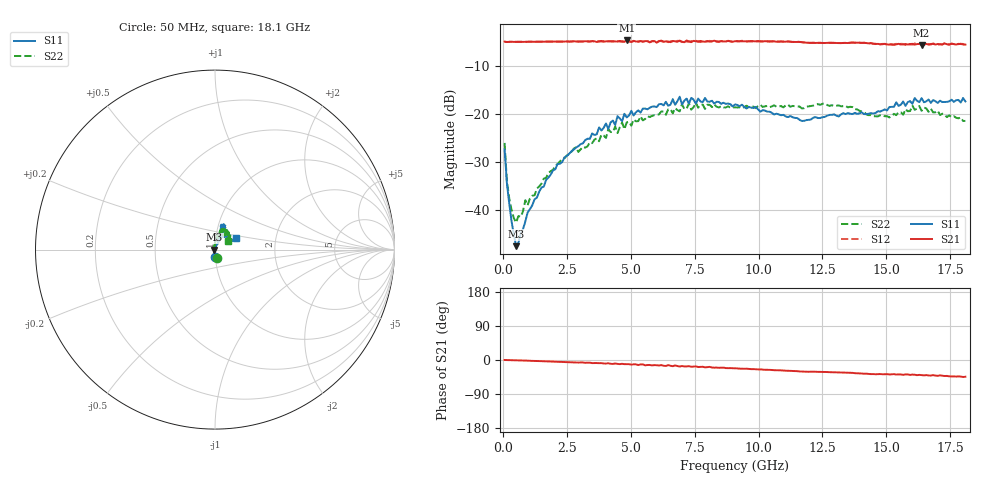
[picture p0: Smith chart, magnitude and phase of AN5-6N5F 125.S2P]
! Network Analyzer HP8720D.06.14 Serial No. US36140669
!  6 Jul 2005  08:33:15
! Frequency  S11  S21  S12  S22
# HZ  S  DB R 50
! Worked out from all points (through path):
!   201 points, 50 MHz to 18.1 GHz, reference 50 ohm
!   highest |S21| = -4.79 dB at 4.833 GHz (marker M1); lowest = -5.7 dB at 16.39 GHz (marker M2)
!   group delay of S21, straight-line fit = 7.04 ps
!   lowest |S11| = -47.6 dB at 501.2 MHz (marker M3), VSWR 1.01, Z = 49.6 - j0.0883 ohm
!   |S11| at or under -10 dB: start of sweep to end of sweep
!   |S22| runs from -42.6 to -17.7 dB; largest |S21 - S12| = 0.023
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5e7  -27.43 -89.4  -5.03 0.0  -5.06 0.1  -26.09 -75.4
1.4025e8  -34.49 -97.5  -5.12 -0.3  -5.11 -0.2  -34.04 -104.6
2.305e8  -38.62 -107.8  -5.09 -0.4  -5.07 -0.4  -37.56 -121.9
5.0125e8  -47.55 -167.7  -5.09 -1.0  -5.07 -1.0  -42.65 -179.7
8.6225e8  -42.41 104.0  -5.07 -1.6  -5.08 -1.6  -37.99 145.1
9.525e8  -40.54 104.0  -5.06 -1.7  -5.06 -1.9  -39.05 129.6
1.6745e9  -33.80 75.6  -5.04 -3.4  -5.03 -3.5  -33.35 100.6
3.1185e9  -26.18 67.9  -4.99 -6.5  -5.02 -6.8  -26.90 89.6
4.021e9  -22.05 67.1  -4.97 -9.4  -5.00 -8.7  -25.05 81.8
4.11125e9  -23.19 66.3  -4.94 -8.6  -4.99 -9.6  -23.22 81.5
4.47225e9  -20.52 62.4  -5.02 -10.3  -4.91 -9.6  -24.04 85.3
4.83325e9  -20.79 71.5  -4.79 -11.0  -4.94 -11.6  -21.82 73.7
6.09675e9  -18.05 67.0  -4.96 -14.4  -4.88 -14.4  -20.16 73.1
6.909e9  -16.48 71.1  -4.81 -17.3  -4.90 -16.0  -19.53 67.6
6.99925e9  -18.11 70.6  -5.04 -15.9  -5.15 -17.4  -18.04 69.4
7.54075e9  -17.93 68.4  -4.96 -16.8  -4.85 -18.9  -17.71 71.3
9.075e9  -18.09 73.1  -4.94 -21.9  -4.92 -22.0  -18.69 59.5
1.21435e10  -20.84 55.0  -5.29 -30.7  -5.25 -30.9  -18.33 60.1
1.512175e10  -18.63 27.9  -5.65 -38.2  -5.52 -37.9  -20.79 59.9
1.602425e10  -17.94 25.1  -5.49 -38.5  -5.65 -40.1  -18.34 50.5
1.638525e10  -16.78 24.0  -5.70 -39.8  -5.48 -39.5  -19.42 45.3
1.81e10  -17.46 29.4  -5.65 -44.1  -5.76 -44.7  -21.52 33.9
